(* Logix 5000 AddOnInstructionDefinition export Banner_TL50Select_PD_v4; software revision 33.00 *)

TYPE Banner_TL50Select_Adv_PD_Seg_v4 :   // Advanced process data set for a TL50 Pro Select Segment.
STRUCT
   Segment_Color_1 : SINT;   // 0 = Green, 1 = Red, 2 = Orange, 3 = Amber, 4 = Yellow, 5 = Lime Green, 6 = Spring Green, 7 = Cyan, 8 = Sky Blue, 9 = Blue, 10 = Violet, 11 = Magenta, 12 = Rose, 13 = White, 14 = Custom, 15 = Custom 2
   Segment_Color_1_Intensity : SINT;   // 0 = High, 1 = Low, 2 = Medium, 3 = Off, 4 = Custom
   Segment_Animation_Type : SINT;   // 0 = Off, 1 = Steady, 2 = Flash, 3 = Two Color, 4 = 50/50, 5 = Intensity Sweep
   Segment_Speed : SINT;   // 0 = Medium, 1 = Fast, 2 = Slow, 3 = Custom
   Segment_Pulse_Pattern : SINT;   // 0 = Normal, 1 = Strobe, 2 = Three Pulse, 3 = SOS, 4 = Random
   Segment_Color_2 : SINT;   // 0 = Green, 1 = Red, 2 = Orange, 3 = Amber, 4 = Yellow, 5 = Lime Green, 6 = Spring Green, 7 = Cyan, 8 = Sky Blue, 9 = Blue, 10 = Violet, 11 = Magenta, 12 = Rose, 13 = White, 14 = Custom, 15 = Custom 2
   Segment_Color_2_Intensity : SINT;   // 0 = High, 1 = Low, 2 = Medium, 3 = Off, 4 = Custom
END_STRUCT
END_TYPE

TYPE Banner_TL50Select_Adv_PDIO_v4 :   // Advanced process data set for a TL50 Pro Select IO-Link unit.
STRUCT
   Segment_1 : Banner_TL50Select_Adv_PD_Seg_v4;   // Advanced process data set for a TL50RGB Segment.
   Segment_2 : Banner_TL50Select_Adv_PD_Seg_v4;   // Advanced process data set for a TL50RGB Segment.
   Segment_3 : Banner_TL50Select_Adv_PD_Seg_v4;   // Advanced process data set for a TL50RGB Segment.
   Segment_4 : Banner_TL50Select_Adv_PD_Seg_v4;   // Advanced process data set for a TL50RGB Segment.
   Audible_State : SINT;   // 0 = Off, 1 = On, 2 = Pulsed, 3 = SOS Pulse
END_STRUCT
END_TYPE

TYPE Banner_TL50Select_Basic_PD_v4 :   // Basic process data set for a TL50 Pro Select IO-Link unit.
STRUCT
   Segment_1 : SINT;   // 0 = Off, 1 = On, 2 = Flash, 3 = Animation Type
   Segment_2 : SINT;   // 0 = Off, 1 = On, 2 = Flash, 3 = Animation Type
   Segment_3 : SINT;   // 0 = Off, 1 = On, 2 = Flash, 3 = Animation Type
   Segment_4 : SINT;   // 0 = Off, 1 = On, 2 = Flash, 3 = Animation Type
   Audible_State : SINT;   // 0 = Off, 1 = On, 2 = Pulsed, 3 = SOS Pulse
END_STRUCT
END_TYPE

TYPE Banner_TL50Select_Level_PD_v4 :   // LeveL process data set for a TL50 Pro Select IO-Link unit.
STRUCT
   Level_Mode_Value : DINT;   // 0 to 65535. 0 = no lights on while 65535 = all lights on.
   Audible_State : SINT;   // 0 = Off, 1 = On, 2 = Pulsed, 3 = SOS Pulse
END_STRUCT
END_TYPE

TYPE Banner_TL50Select_PDIO_v4 :   // Process data for a Banner TL50 Pro Select unit. This includes four process data types.
STRUCT
   Basic_PD : Banner_TL50Select_Basic_PD_v4;
   Advanced_PD : Banner_TL50Select_Adv_PDIO_v4;
   Run_PD : Banner_TL50Select_Run_PD_v4;
   Level_PD : Banner_TL50Select_Level_PD_v4;
   ReverseAdv_PD : Banner_TL50Select_Adv_PDIO_v4;
   Transfer_Data : SINT[14];   // Data array to send teh correct state of the process data output to the IO-Link master.
END_STRUCT
END_TYPE

TYPE Banner_TL50Select_Run_PD_v4 :   // Run mode process data set for a TL50 Pro Select IO-Link unit.
STRUCT
   Animation : SINT;   // 0 = Off, 1 = Steady, 2 = Flash, 3 = Two Color, 4 = 50/50, 5 = Intesnity Sweep, 6 = Scroll, 7 = Bounce, 8 = Color Spectrum, 9 = Demo
   Color_1 : SINT;   // 0 = Green, 1 = Red, 2 = Orange, 3 = Amber, 4 = Yellow, 5 = Lime Green, 6 = Spring Green, 7 = Cyan, 8 = Sky Blue, 9 = Blue, 10 = Violet, 11 = Magenta, 12 = Rose, 13 = White, 14 = Custom, 15 = Custom 2
   Color_1_Intensity : SINT;   // 0 = High, 1 = Low, 2 = Medium, 3 = Off, 4 = Custom
   Speed : SINT;   // 0 = Medium, 1 = Fast, 2 = Slow, 3 = Custom
   Pulse_Pattern : SINT;   // 0 = Normal, 1 = Strobe, 2 = Three Pulse, 3 = SOS, 4 = Random
   Color_2 : SINT;   // 0 = Green, 1 = Red, 2 = Orange, 3 = Amber, 4 = Yellow, 5 = Lime Green, 6 = Spring Green, 7 = Cyan, 8 = Sky Blue, 9 = Blue, 10 = Violet, 11 = Magenta, 12 = Rose, 13 = White, 14 = Custom, 15 = Custom 2
   Color_2_Intensity : SINT;   // 0 = High, 1 = Low, 2 = Medium, 3 = Off, 4 = Custom
   Direction : SINT;   // 0 = Up, 1 = Down
   Audible_State : SINT;   // 0 = Off, 1 = On, 2 = Pulsed, 3 = SOS Pulse
END_STRUCT
END_TYPE

ADD_ON_INSTRUCTION Banner_TL50Select_Adv_PD_v4   (* revision 4.0, vendor Banner Engineering *)
// AOI converts the Advanced process and places it into the correct bytes for transfer to the IO-Link master.
VAR_IN_OUT
   TL50_Pro_Segment : Banner_TL50Select_Adv_PD_Seg_v4; {required}
   Data_Byte_1 : SINT; {required}
   Data_Byte_2 : SINT; {required}
   Data_Byte_3 : SINT; {required}
END_VAR

ROUTINE Logic   (* ladder *)
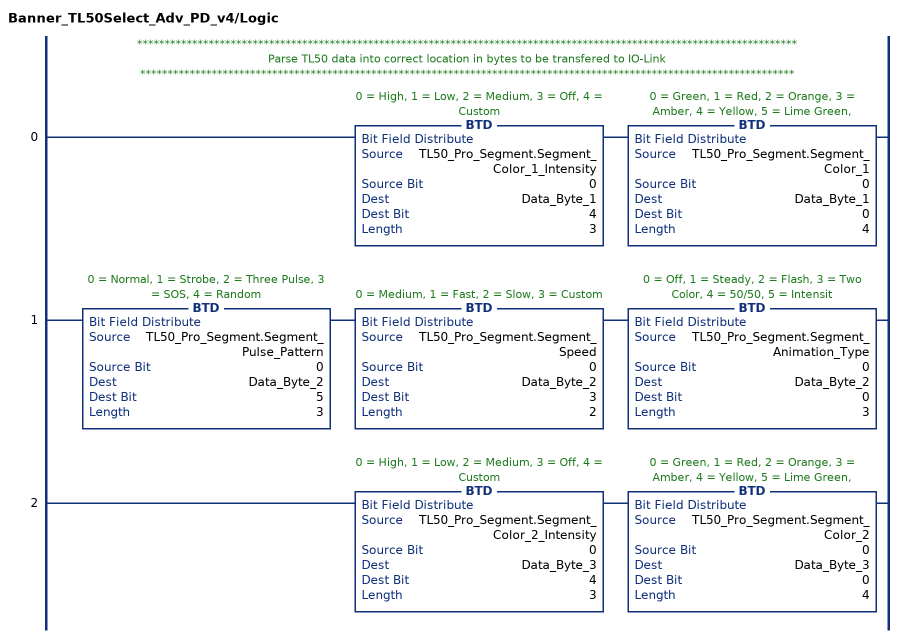
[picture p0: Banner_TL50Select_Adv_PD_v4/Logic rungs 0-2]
   // ************************************************************************************************************************
   // Parse TL50 data into correct location in bytes to be transfered to IO-Link
   // ***********************************************************************************************************************
   0: BTD(TL50_Pro_Segment.Segment_Color_1_Intensity,0,Data_Byte_1,4,3)BTD(TL50_Pro_Segment.Segment_Color_1,0,Data_Byte_1,0,4);
   1: BTD(TL50_Pro_Segment.Segment_Pulse_Pattern,0,Data_Byte_2,5,3)BTD(TL50_Pro_Segment.Segment_Speed,0,Data_Byte_2,3,2)BTD(TL50_Pro_Segment.Segment_Animation_Type,0,Data_Byte_2,0,3);
   2: BTD(TL50_Pro_Segment.Segment_Color_2_Intensity,0,Data_Byte_3,4,3)BTD(TL50_Pro_Segment.Segment_Color_2,0,Data_Byte_3,0,4);
END_ROUTINE
END_ADD_ON_INSTRUCTION

ADD_ON_INSTRUCTION Banner_TL50Select_PD_v4   (* revision 4.0, vendor Banner Engineering *)
// Takes the raw SINT information and converts that data into actual information.
VAR_IN_OUT
   PD : Banner_TL50Select_PDIO_v4; {required}
END_VAR
VAR_INPUT
   Byte_Swap : BOOL; {required}   // Swap the LSB and the MSB with each other.
   Operation_Mode : INT; {required}   // 0 = Basic, 1 = Advanced, 2 = Run, 3 = Level
END_VAR
VAR
   Temp_Measurement : DINT; {access None}
   Data_Byte : SINT[14]; {access None}
   Temp_Data : SINT[14]; {access None}
   AOI_Status : Banner_TL50Select_Adv_PD_v4[4]; {access None}
   Control : CONTROL[4]; {access None}
END_VAR

ROUTINE Logic   (* ladder *)
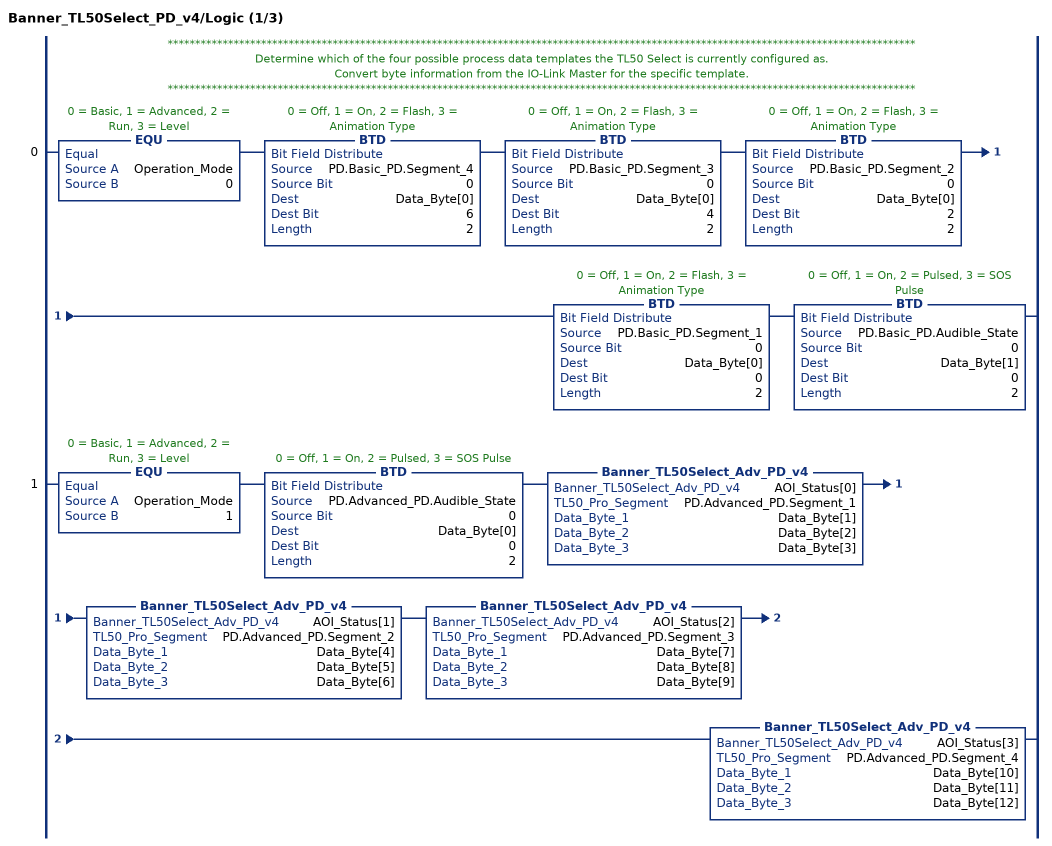
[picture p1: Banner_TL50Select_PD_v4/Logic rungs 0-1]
   // ****************************************************************************************************************************************
   // Determine which of the four possible process data templates the TL50 Select is currently configured as.
   // Convert byte information from the IO-Link Master for the specific template.
   // ****************************************************************************************************************************************
   0: EQU(Operation_Mode,0)BTD(PD.Basic_PD.Segment_4,0,Data_Byte[0],6,2)BTD(PD.Basic_PD.Segment_3,0,Data_Byte[0],4,2)BTD(PD.Basic_PD.Segment_2,0,Data_Byte[0],2,2)BTD(PD.Basic_PD.Segment_1,0,Data_Byte[0],0,2)BTD(PD.Basic_PD.Audible_State,0,Data_Byte[1],0,2);
   1: EQU(Operation_Mode,1)BTD(PD.Advanced_PD.Audible_State,0,Data_Byte[0],0,2)Banner_TL50Select_Adv_PD_v4(AOI_Status[0],PD.Advanced_PD.Segment_1,Data_Byte[1],Data_Byte[2],Data_Byte[3])Banner_TL50Select_Adv_PD_v4(AOI_Status[1],PD.Advanced_PD.Segment_2,Data_Byte[4],Data_Byte[5],Data_Byte[6])Banner_TL50Select_Adv_PD_v4(AOI_Status[2],PD.Advanced_PD.Segment_3,Data_Byte[7],Data_Byte[8],Data_Byte[9])Banner_TL50Select_Adv_PD_v4(AOI_Status[3],PD.Advanced_PD.Segment_4,Data_Byte[10],Data_Byte[11],Data_Byte[12]);
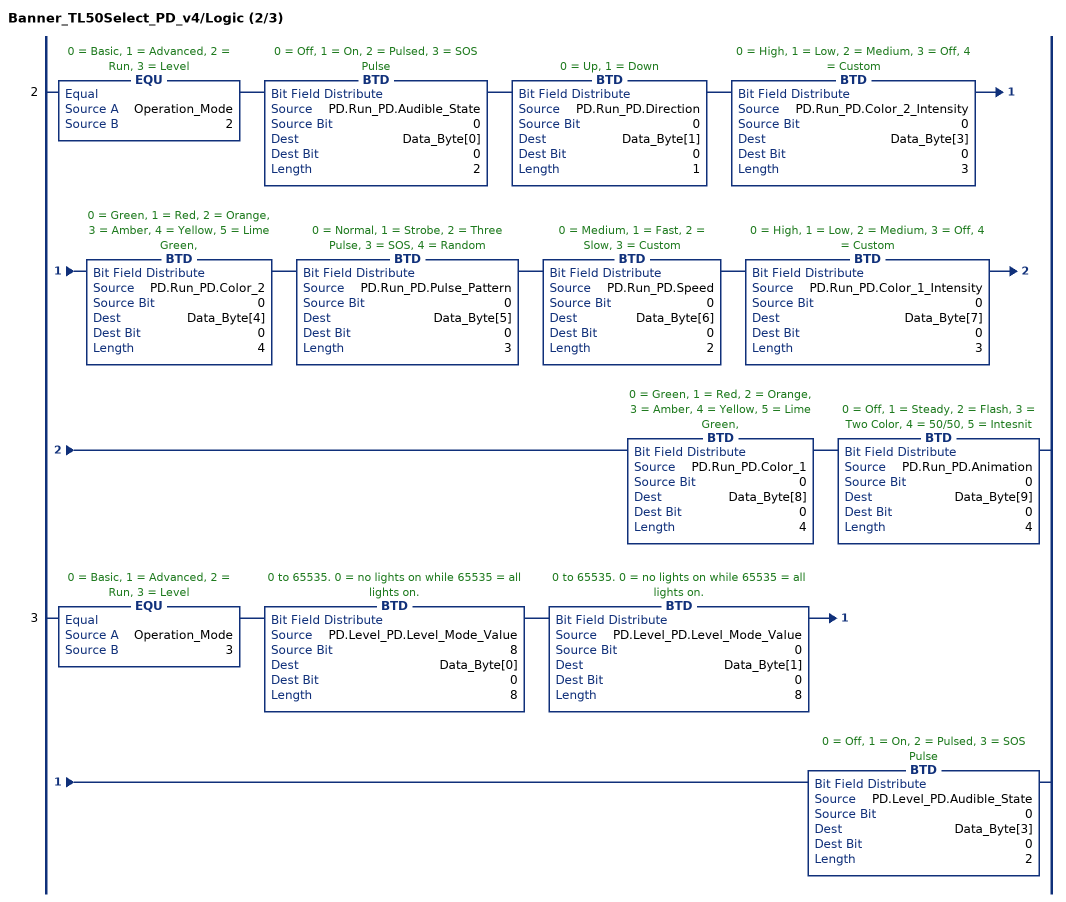
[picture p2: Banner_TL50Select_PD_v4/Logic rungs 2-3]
   2: EQU(Operation_Mode,2)BTD(PD.Run_PD.Audible_State,0,Data_Byte[0],0,2)BTD(PD.Run_PD.Direction,0,Data_Byte[1],0,1)BTD(PD.Run_PD.Color_2_Intensity,0,Data_Byte[3],0,3)BTD(PD.Run_PD.Color_2,0,Data_Byte[4],0,4)BTD(PD.Run_PD.Pulse_Pattern,0,Data_Byte[5],0,3)BTD(PD.Run_PD.Speed,0,Data_Byte[6],0,2)BTD(PD.Run_PD.Color_1_Intensity,0,Data_Byte[7],0,3)BTD(PD.Run_PD.Color_1,0,Data_Byte[8],0,4)BTD(PD.Run_PD.Animation,0,Data_Byte[9],0,4);
   3: EQU(Operation_Mode,3)BTD(PD.Level_PD.Level_Mode_Value,8,Data_Byte[0],0,8)BTD(PD.Level_PD.Level_Mode_Value,0,Data_Byte[1],0,8)BTD(PD.Level_PD.Audible_State,0,Data_Byte[3],0,2);
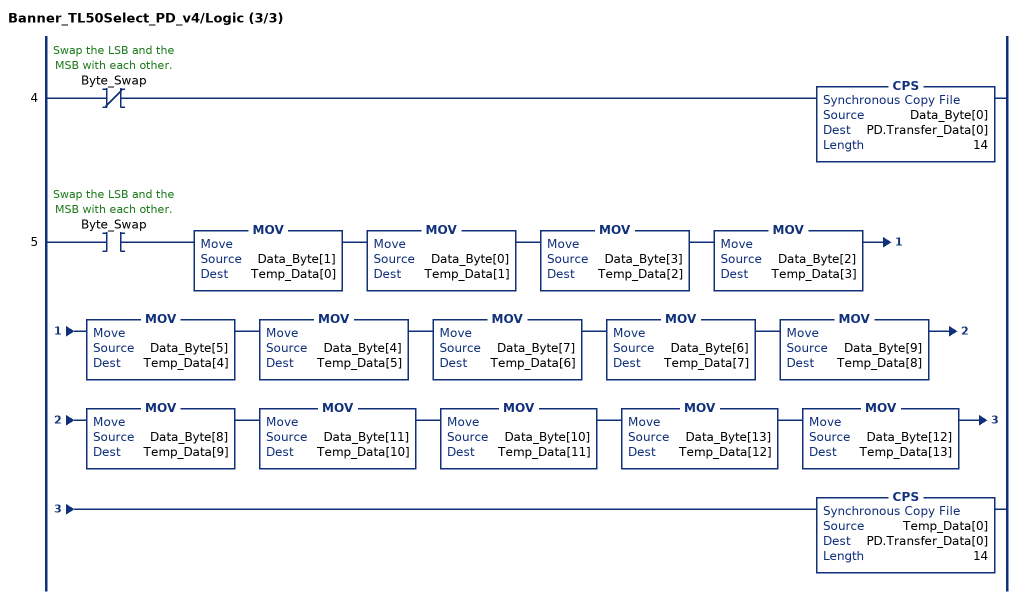
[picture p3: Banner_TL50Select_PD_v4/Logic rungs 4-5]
   4: XIO(Byte_Swap)CPS(Data_Byte[0],PD.Transfer_Data[0],14);
   5: XIC(Byte_Swap)MOV(Data_Byte[1],Temp_Data[0])MOV(Data_Byte[0],Temp_Data[1])MOV(Data_Byte[3],Temp_Data[2])MOV(Data_Byte[2],Temp_Data[3])MOV(Data_Byte[5],Temp_Data[4])MOV(Data_Byte[4],Temp_Data[5])MOV(Data_Byte[7],Temp_Data[6])MOV(Data_Byte[6],Temp_Data[7])MOV(Data_Byte[9],Temp_Data[8])MOV(Data_Byte[8],Temp_Data[9])MOV(Data_Byte[11],Temp_Data[10])MOV(Data_Byte[10],Temp_Data[11])MOV(Data_Byte[13],Temp_Data[12])MOV(Data_Byte[12],Temp_Data[13])CPS(Temp_Data[0],PD.Transfer_Data[0],14);
END_ROUTINE
END_ADD_ON_INSTRUCTION
